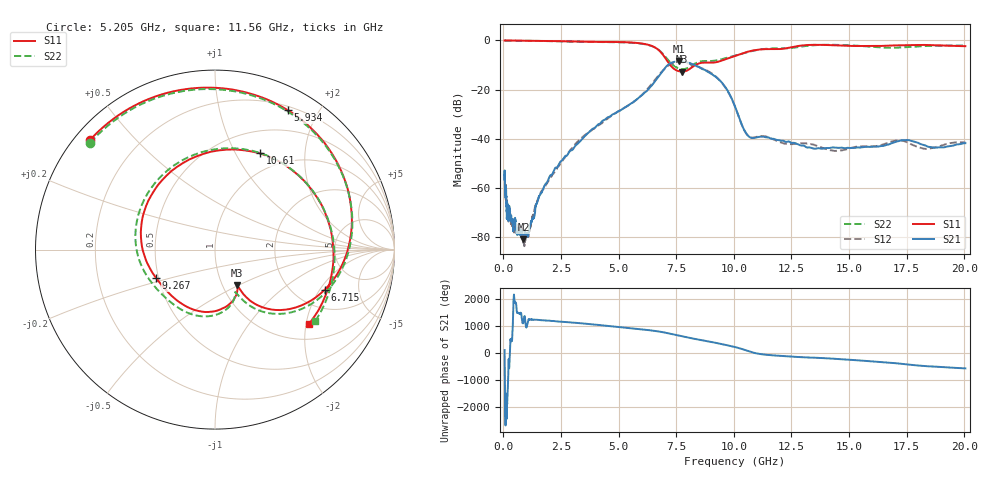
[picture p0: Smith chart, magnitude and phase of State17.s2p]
# Hz S DB R 50
!freq MagS11 AngS11 MagS21 AngS21 MagS12 AngS12 MagS22 AngS22
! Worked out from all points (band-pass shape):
!   1601 points, 50 MHz to 20.05 GHz, reference 50 ohm
!   highest |S21| = -8.50 dB at 7.599 GHz (marker M1); lowest = -80.9 dB at 868.4 MHz (marker M2)
!   |S21| within 3 dB of the highest: 6.985 GHz to 8.604 GHz (1.619 GHz wide, 20.8 % of centre)
!   lowest |S11| = -12.7 dB at 7.742 GHz (marker M3), VSWR 1.61, Z = 58.5 - j24.4 ohm
!   |S11| at or under -10 dB: 7.238 GHz to 8.333 GHz (1.095 GHz wide, 14.1 % of centre)
!   |S22| runs from -11.6 to 0.0 dB; largest |S21 - S12| = 0.021
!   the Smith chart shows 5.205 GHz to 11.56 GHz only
!   S11 on the Smith chart (normalised r, x): 5.205 GHz: 0.04, +0.38; 5.934 GHz: 0.24, +1.62; 6.715 GHz: 2.88, -2.22; 9.267 GHz: 0.49, -0.18; 10.61 GHz: 0.76, +1.26; 11.56 GHz: 1.40, -2.08
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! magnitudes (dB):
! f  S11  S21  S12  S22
! 50 MHz  0.0  -54.2  -53.0  0.0
! 69.79 MHz  0.0  -60.8  -59.8  0.0
! 115.7 MHz  0.0  -60.8  -64.4  0.0
! 135.9 MHz  0.0  -67.8  -65.9  0.0
! 148.2 MHz  0.0  -71.9  -66.7  0.0
! 160.3 MHz  0.0  -66.2  -69.7  0.0
! 174.1 MHz  0.0  -72.1  -69.2  0.0
! 369.6 MHz  0.0  -73.1  -75.5  0.0
! 868.4 MHz  -0.1  -80.9  -82.3  -0.1
! 1.005 GHz  -0.1  -78.5  -78.3  -0.1
! 2.722 GHz  -0.3  -47.0  -46.8  -0.4
! 5.205 GHz  -0.7  -27.6  -27.6  -0.8
! 5.934 GHz  -1.1  -22.8  -22.8  -1.2
! 6.715 GHz  -3.7  -14.8  -14.4  -3.6
! 7.402 GHz  -11.5  -8.7  -9.1  -10.3
! 7.599 GHz  -12.5  -8.5  -8.8  -11.3
! 7.742 GHz  -12.7  -8.5  -8.9  -11.6
! 9.267 GHz  -8.8  -15.2  -15.1  -8.1
! 10.61 GHz  -4.6  -38.7  -38.5  -4.7
! 11.56 GHz  -3.5  -39.6  -39.6  -3.3
! 14.42 GHz  -2.0  -43.5  -44.9  -1.8
! 20.05 GHz  -2.3  -41.7  -41.4  -2.1
